PROGRAM FAST
VAR
	iCounter AT %Q* 		: UDINT;			// link to a digital/analogue output terminal
	iTest AT %I*	 		: UDINT;			// link to a digital/analogue output terminal

	(* ******************* EtherCAT Frame ***************************** *)
	fbEtherCATFrameDiag		: FB_EtherCATFrameDiag; // frame diagnostic
	wFrmXWcState AT %I*		: WORD; 			// link to task related ethercat frame state (Frm1WcState)
	wReqZeroMask			: WORD := 16#FFFF; 	// clear bit to ignore datagram error of Frm1WcState
	bFrameWcStateOK			: BOOL;				// this frame is OK
END_VAR

iCounter := iCounter + 1;

(*************************************** Frame Diag *********************************************)
fbEtherCATFrameDiag(
	wFrmXWcState 	:= wFrmXWcState,
	wReqZeroMask 	:= wReqZeroMask,
	bFrameWcStateOK	=> bFrameWcStateOK
);

END_PROGRAM
